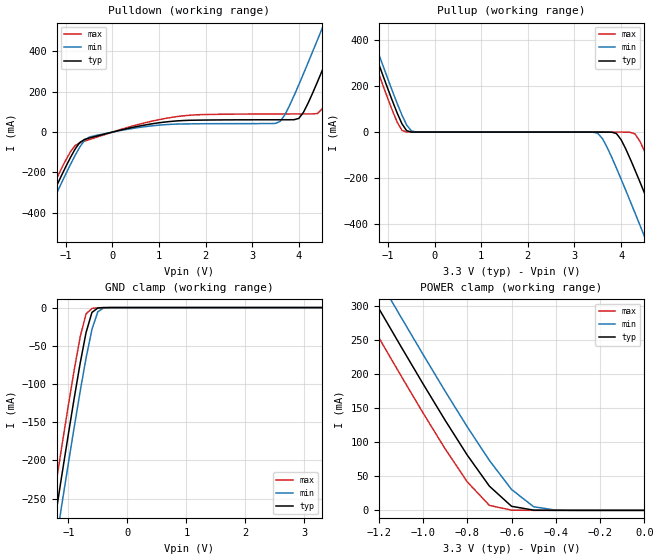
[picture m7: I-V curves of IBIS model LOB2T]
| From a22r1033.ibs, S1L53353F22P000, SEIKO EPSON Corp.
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[Model]   LOB2T
Model_type   Output
Polarity   Non-Inverting
|   typ   min   max
C_comp   5.0pF   4.0pF   6.0pF
|   typ   min   max
[Voltage range]   3.3   3.0   3.6
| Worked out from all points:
|   slope of the pulldown table from 0 to 0.495 V, typ, clamps not added: 18.9 ohm
|   GND clamp passes 1 mA (typ) near -0.51 V on its own axis
|   POWER clamp passes 1 mA (typ) near -0.51 V on its own axis
[Pulldown]
|   Voltage   I(typ)   I(min)   I(max)
-3.3V     -1.344A    -1.379A    -1.31A
-1.8V     -569.4mA   -606.5mA   -533mA
-1.6V     -467.5mA   -504.9mA   -431mA
-900mV    -125.3mA   -160mA     -97.15mA
-500mV    -29.58mA   -25.14mA   -37.43mA
1.4V      55.64mA    39.77mA    77.15mA
3.6V      61.14mA    53.33mA    89.83mA
4V        67.97mA    235.6mA    89.96mA
4.5V      304.8mA    514.4mA    115.4mA
4.9V      531mA      743.5mA    321.7mA
5.3V      761.4mA    974.8mA    549.5mA
6.6V      1.52A      1.732A     1.307A
[Pullup]
|   Voltage   I(typ)   I(min)   I(max)
-3.3V     1.514A     1.553A     1.476A
-1.5V     467mA      509.6mA    424.7mA
-1.4V     409.9mA    452.7mA    367.4mA
-800mV    81.11mA    122.6mA    41.82mA
-600mV    5.969mA    30.7mA     281.7uA
3.5V      -254.2nA   -5.399mA   -6.778nA
3.9V      -6.318mA   -156.3mA   -836.6nA
4.3V      -165.9mA   -352.4mA   -8.315mA
4.5V      -264.1mA   -453mA     -81.32mA
4.9V      -465.8mA   -656.6mA   -276.1mA
5.3V      -670.6mA   -861.9mA   -479.7mA
6.6V      -1.343A    -1.534A    -1.153A
[GND_clamp]
|   Voltage   I(typ)   I(min)   I(max)
-3.3V     -1.343A    -1.379A    -1.309A
-1.3V     -314.1mA   -352.4mA   -276.2mA
-1.2V     -264.1mA   -302.5mA   -226.1mA
-1.1V     -214.6mA   -253.1mA   -176.6mA
-1V       -165.9mA   -204.2mA   -128.1mA
-900mV    -118.4mA   -156.3mA   -81.33mA
-800mV    -73.08mA   -109.9mA   -38.6mA
-700mV    -32.75mA   -66.18mA   -8.318mA
-600mV    -6.318mA   -28.41mA   -1.129mA
-500mV    -586.9uA   -5.399mA   -239.5uA
-400mV    -56.77uA   -404.4uA   -18.72uA
3.3V      7.178nA    15.7uA     6.022nA
[POWER_clamp]
|   Voltage   I(typ)   I(min)   I(max)
-3.3V     1.514A     1.553A     1.476A
-1.3V     353.1mA    396.1mA    310.4mA
-1.2V     296.7mA    339.9mA    253.9mA
-1.1V     240.9mA    284.1mA    198mA
-1V       185.9mA    229mA      143.2mA
-900mV    132.3mA    175mA      90.33mA
-800mV    81.11mA    122.6mA    41.82mA
-700mV    35.52mA    73.27mA    7.314mA
-600mV    5.969mA    30.7mA     281.7uA
-500mV    284.1uA    5.285mA    30.01uA
-400mV    15.7uA     326.5uA    2.385uA
0V        7.178nA    15.84nA    7.223nA
[Ramp]
|   V_typ   V_min   V_max
dV/dt_r   1.98/0.83n   1.80/1.10n   2.16/0.56n
dV/dt_f   1.98/0.71n   1.80/0.94n   2.16/0.49n
R_load = 5000
